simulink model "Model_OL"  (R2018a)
settings: Solver=ode15s  StartTime=0.0  StopTime=tsim  RelTol=1e-5
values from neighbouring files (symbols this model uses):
  C = Fc*cpc/(Fh*cph)    [calcblock.m]    (also in eNTU.m = m.c*cp.c/(m.h*cp.h); Main.m = [zeros(1,2*N-1),1]; Main_OL.m = [zeros(1,2*N-1),1]; testfun.m = mc*cpc/(mh*cph))
  d0 = [Fh, Tcin, Thin]    [Main.m]    (also in Main_OL.m; runTestCalcBlk.m; runTransf.m = [Fh; Tcin; U0; Ffeed0; m0; Tfeed0]; runTransfOL.m)
  d_step = [Fh, Tcin, Thin]    [Main.m]    (also in Main_OL.m = [Fh, Tcin+0, Thin]; runTestCalcBlk.m)
  d_tstep = [1000; 1000;2000]    [Main.m]    (also in Main_OL.m = 300; runTestCalcBlk.m = 300; runTransf.m = [500; 50000; 70000; 130000; 50000; 50000]; runTransfOL.m = [500 5000 7000 13000])
  dFc = dist(i)    [Main_OL.m]    (also in Main.m = 0; runTransfOL.m = -0.5)
  Fc0 = 5    [Main.m]    (also in Main_OL.m; runTestCalcBlk.m; runTransf.m; runTransfOL.m)
  nd = size(d0,2)    [Main.m]    (also in Main_OL.m; runTestCalcBlk.m; runTransf.m = size(d0,1); runTransfOL.m)
  np = size(p,2)    [Main.m]    (also in Main_OL.m; runH2Psim.m = length(param); runTestCalcBlk.m; runTransf.m)
  nu = 1    [Main.m]    (also in Main_OL.m; runH2Psim.m = length(u0); runTestCalcBlk.m; runTransf.m)
  nx = size(x0,1)    [Main.m]    (also in Main_OL.m; H2P_Turbine_driven.m = param(end); runTD.m = length(x0); H2P_Boiler_driven.m = param(end))
  p = [N, Fc0, rhoc, rhoh,U,A,cpc,cph]    [Main.m]    (also in Main_OL.m; runTestCalcBlk.m; NonlinearMap.m = [U;A;Fc(i);Fh;cpc;cph;Tcin;Thin]; runTransf.m = [N, Fc0, rhoc, rhoh, U0, A,cpc,cph])
  tstep = 100    [Main_OL.m]    (also in Main.m; runTransf.m = 10000; runTransfOL.m)
  x0 = [Tcend(1:N)'; Thend(1:N)']    [Main.m]    (also in Main_OL.m; runTD.m = [TE0;TD0;TSh0;MD0; MSh0;w0;TA0;0;0;0;0;0;0;0;0;0]; runBD.m = [TE0;TD0;TSh0;MD0; MSh0;w0;TA0;0;0;0;0;0;0;0;0;0]; runFP.m = [TE0;TD0;TSh0;MD0; MSh0;w0;TA0;0;0;0;0;0;0;0])
undefined symbols (not defined in the file or in its folder): HEXode

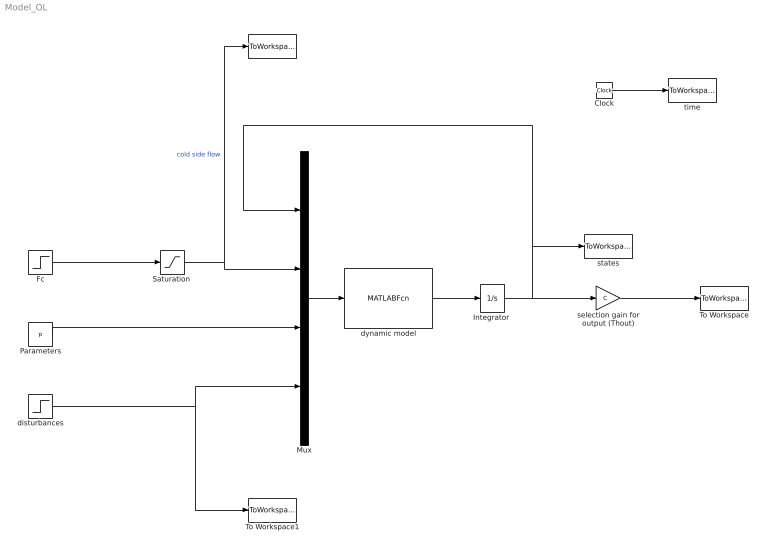
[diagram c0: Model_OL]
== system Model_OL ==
  " " : ToWorkspace  VariableName=uc  SampleTime=-1
  Clock : Clock
  Fc : Step  Time=tstep  Before=Fc0  After=Fc0+dFc  SampleTime=0
  "Integrator " : Integrator  InitialCondition=x0
  Mux : Mux
  Parameters : Constant  Value=p
  "Saturation " : Saturate  UpperLimit=inf  LowerLimit=0
  To Workspace : ToWorkspace  VariableName=Thout  SampleTime=-1
  To Workspace1 : ToWorkspace  VariableName=dsim  SampleTime=-1
  disturbances : Step  Time=d_tstep  Before=d0  After=d_step  SampleTime=0
  dynamic model : MATLABFcn  MATLABFcn=HEXode(u(1:nx),u(nx+1:nx+nu),u(nx+nu+1:nx+nu+np),u(nx+nu+np+1:nx+nu+np+nd))  OutputDimensions=nx  Output1D=off
  selection gain for output (Thout) : Gain  Gain=C  Multiplication=Matrix(K*u)
  states : ToWorkspace  VariableName=T  SampleTime=-1
  time : ToWorkspace  VariableName=t  SampleTime=-1
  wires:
  dynamic model/1 -> "Integrator "/1
  "Integrator "/1 -> selection gain for output (Thout)/1, states/1, Mux/1
  Mux/1 -> dynamic model/1
  Clock/1 -> time/1
  Parameters/1 -> Mux/3
  disturbances/1 -> Mux/4, To Workspace1/1
  "Saturation "/1 -> Mux/2, " "/1  "cold side flow"
  selection gain for output (Thout)/1 -> To Workspace/1
  Fc/1 -> "Saturation "/1
